| TEXAS INSTRUMENTS INCORPORATED
| Standard Linear and Logic Group
| IBIS Model of PCA9546A
| 4-CHANNEL I2C AND SMBus SWITCH WITH RESET FUNCTION
| This file contains package information for the following:
|  QFN 16-pin (RGY) package as [Component] PCA9546A_RGY
|  SOIC 16-pin (D) package as [Component] PCA9546A_D
|  SOIC 16-pin (DW) package as [Component] PCA9546A_DW
|  TSSOP 16-pin (PW) package as [Component] PCA9546A_PW
|  TVSOP 16-pin (DGV) package as [Component] PCA9546A_DGV
| This device can be powered at the following Vccs:
|  5 volt Vcc
|  3.3 volt Vcc
|  2.5 volt Vcc
| This file provides unique models under the [Model Selector] for each Vcc.
| For operation at a specific Vcc, select the appropriate model after each
| [Model Selector] keyword.
[IBIS Ver]   3.2
[Comment char]  |_char
[File Name]   pca9546a.ibs
[File Rev]   1.1 | a_die
[Date]   May 2, 2007
[Source]   Data created from TI-SPICE simulations at TI-SLL.
[Notes]   The following is an IBIS list for the PCA9546A.
   Please contact sllibis@ti.com with questions and
   comments concerning SLL IBIS models.
   - FILE REV HISTORY
   - 1.1 Release IBIS file on 5/4/07
   - Power clamp data has been deleted in all models except
   SDA terminator models as there is no power-clamp diode.
   - Non-monotonic data due to FET characteristics.
[Disclaimer] Property of Texas Instruments Incorporated.  Unauthorized
   reproduction and/or distribution is strictly prohibited.
   This product is protected under copyright law.
   Created  2007, (C) Copyright  2007, Texas Instruments
   Incorporated, All Rights Reserved
   UNLESS THERE IS A SIGNED, WRITTEN AGREEMENT TO THE
   CONTRARY, TEXAS INSTRUMENTS (TI) IS PROVIDING THE IBIS
   MODELS  AND WITHOUT ANY WARRANTY, EXPRESSED OR
   IMPLIED.  TI assumes no liability for:
   1) the accuracy of the IBIS models provided to your
   company;
   2) the proper functioning of these IBIS Models in your
   design or for any resulting applications; or
   3) infringement of patents, copyrights or intellectual
   property rights resulting from your use of these IBIS
   models.
   TI provides IBIS Models as a service to our customers.
   You and your company shall not distribute, sell or give
   these models to anyone else without prior written
   permission from TI.
   TI reserves the right to make changes to our products or
   to discontinue any semiconductor product or service
   without notice, and advises our customers to obtain the
   latest version of relevant information to verify, before
   placing orders, that the information being relied on is
   current.
   Please be aware that your receipt and use of the IBIS
   information provided shall serve as acceptance of these
   terms and conditions.  If you do not accept these terms,
   you should return or destroy the IBIS models and any
   other accompanying information immediately.
| Component PCA9546A_RGY 16-PIN QFN
[Component]   PCA9546A_RGY
[Manufacturer]   Texas Instruments, Inc.
[Package]
|   typ   min   max
R_pkg   3.900e-02   3.700e-02   4.200e-02
L_pkg   8.860e-10   8.430e-10   9.330e-10
C_pkg   3.270e-13   3.140e-13   3.360e-13
[Pin]   signal_name   model_name   R_pin   L_pin   C_pin
1   A0   PCA9546_A   4.100e-02   9.250e-10   3.140e-13
2   A1   PCA9546_A   4.000e-02   9.000e-10   3.260e-13
3   NRESET   NC   3.900e-02   8.820e-10   3.330e-13
4   SD0   PCA9546_SDX   4.100e-02   9.150e-10   3.300e-13
5   SC0   PCA9546_SCX   4.000e-02   9.000e-10   3.300e-13
6   SD1   PCA9546_SDX   4.000e-02   8.910e-10   3.290e-13
7   SC1   PCA9546_SCX   4.100e-02   9.240e-10   3.300e-13
8   GND   GND   4.200e-02   9.330e-10   3.360e-13
9   SD2   PCA9546_SDX   3.900e-02   8.850e-10   3.250e-13
10   SC2   PCA9546_SCX   3.700e-02   8.430e-10   3.210e-13
11   SD3   PCA9546_SDX   3.900e-02   8.730e-10   3.310e-13
12   SC3   PCA9546_SCX   3.800e-02   8.550e-10   3.250e-13
13   A2   PCA9546_A   3.800e-02   8.530e-10   3.260e-13
14   SCL   PCA9546_SCL   3.800e-02   8.570e-10   3.270e-13
15   SDA   PCA9546_SDA   3.800e-02   8.540e-10   3.250e-13
16   VCC   POWER   3.900e-02   8.850e-10   3.190e-13
| Component PCA9546A_D 16-PIN SOIC
[Component]   PCA9546A_D
[Manufacturer]   Texas Instruments, Inc.
[Package]
|   typ   min   max
R_pkg   3.900e-02   2.800e-02   4.900e-02
L_pkg   3.453e-09   2.350e-09   4.375e-09
C_pkg   5.210e-13   2.540e-13   7.080e-13
[Pin]   signal_name   model_name   R_pin   L_pin   C_pin
1   A0   PCA9546_A   4.200e-02   4.336e-09   7.030e-13
2   A1   PCA9546_A   4.900e-02   3.778e-09   6.340e-13
3   NRESET   NC   2.800e-02   3.449e-09   5.180e-13
4   SD0   PCA9546_SDX   2.900e-02   2.393e-09   2.540e-13
5   SC0   PCA9546_SCX   2.800e-02   2.350e-09   2.640e-13
6   SD1   PCA9546_SDX   4.800e-02   3.312e-09   4.830e-13
7   SC1   PCA9546_SCX   4.300e-02   3.629e-09   6.040e-13
8   GND   GND   4.400e-02   4.375e-09   7.080e-13
9   SD2   PCA9546_SDX   4.200e-02   4.336e-09   7.030e-13
10   SC2   PCA9546_SCX   4.900e-02   3.778e-09   6.340e-13
11   SD3   PCA9546_SDX   2.800e-02   3.449e-09   5.180e-13
12   SC3   PCA9546_SCX   2.900e-02   2.393e-09   2.550e-13
13   A2   PCA9546_A   2.800e-02   2.350e-09   2.640e-13
14   SCL   PCA9546_SCL   4.800e-02   3.312e-09   4.830e-13
15   SDA   PCA9546_SDA   4.300e-02   3.629e-09   6.040e-13
16   VCC   POWER   4.400e-02   4.375e-09   7.080e-13
| Component PCA9546A_DW 16-PIN SOIC
[Component]   PCA9546A_DW
[Manufacturer]   Texas Instruments, Inc.
[Package]
|   typ   min   max
R_pkg   4.600e-02   3.400e-02   5.700e-02
L_pkg   4.858e-09   3.987e-09   6.214e-09
C_pkg   7.150e-13   5.020e-13   1.046e-12
[Pin]   signal_name   model_name   R_pin   L_pin   C_pin
1   A0   PCA9546_A   5.700e-02   6.214e-09   1.026e-12
2   A1   PCA9546_A   5.500e-02   5.236e-09   8.180e-13
3   NRESET   NC   3.400e-02   3.987e-09   7.230e-13
4   SD0   PCA9546_SDX   3.600e-02   3.996e-09   7.260e-13
5   SC0   PCA9546_SCX   3.600e-02   3.996e-09   7.260e-13
6   SD1   PCA9546_SDX   3.400e-02   3.987e-09   7.040e-13
7   SC1   PCA9546_SCX   5.500e-02   5.236e-09   8.180e-13
8   GND   GND   5.700e-02   6.214e-09   1.046e-12
9   SD2   PCA9546_SDX   5.700e-02   6.214e-09   8.270e-13
10   SC2   PCA9546_SCX   5.500e-02   5.236e-09   5.970e-13
11   SD3   PCA9546_SDX   3.400e-02   3.987e-09   5.020e-13
12   SC3   PCA9546_SCX   3.600e-02   3.996e-09   5.050e-13
13   A2   PCA9546_A   3.600e-02   3.996e-09   5.050e-13
14   SCL   PCA9546_SCL   3.400e-02   3.987e-09   5.020e-13
15   SDA   PCA9546_SDA   5.500e-02   5.236e-09   5.970e-13
16   VCC   POWER   5.700e-02   6.214e-09   8.270e-13
| Component PCA9546A_PW 16-PIN TSSOP
[Component]   PCA9546A_PW
[Manufacturer]   Texas Instruments, Inc.
[Package]
|   typ   min   max
R_pkg   4.500e-02   3.800e-02   5.100e-02
L_pkg   2.593e-09   2.447e-09   3.080e-09
C_pkg   2.810e-13   2.430e-13   3.770e-13
[Pin]   signal_name   model_name   R_pin   L_pin   C_pin
1   A0   PCA9546_A   4.000e-02   3.080e-09   3.770e-13
2   A1   PCA9546_A   3.800e-02   2.458e-09   2.810e-13
3   NRESET   NC   5.100e-02   2.512e-09   2.550e-13
4   SD0   PCA9546_SDX   5.100e-02   2.447e-09   2.430e-13
5   SC0   PCA9546_SCX   5.100e-02   2.447e-09   2.430e-13
6   SD1   PCA9546_SDX   5.100e-02   2.512e-09   2.550e-13
7   SC1   PCA9546_SCX   3.800e-02   2.458e-09   2.810e-13
8   GND   GND   4.000e-02   3.080e-09   3.770e-13
9   SD2   PCA9546_SDX   3.900e-02   2.832e-09   3.160e-13
10   SC2   PCA9546_SCX   3.800e-02   2.460e-09   2.790e-13
11   SD3   PCA9546_SDX   5.100e-02   2.512e-09   2.550e-13
12   SC3   PCA9546_SCX   5.100e-02   2.447e-09   2.430e-13
13   A2   PCA9546_A   5.100e-02   2.447e-09   2.430e-13
14   SCL   PCA9546_SCL   5.100e-02   2.512e-09   2.550e-13
15   SDA   PCA9546_SDA   3.800e-02   2.459e-09   2.790e-13
16   VCC   POWER   3.900e-02   2.832e-09   3.160e-13
| Component PCA9546A_DGV 16-PIN TVSOP
[Component]   PCA9546A_DGV
[Manufacturer]   Texas Instruments, Inc.
[Package]
|   typ   min   max
R_pkg   3.900e-02   3.300e-02   4.500e-02
L_pkg   2.543e-09   2.320e-09   2.938e-09
C_pkg   3.860e-13   3.340e-13   4.490e-13
[Pin]   signal_name   model_name   R_pin   L_pin   C_pin
1   A0   PCA9546_A   3.500e-02   2.907e-09   4.170e-13
2   A1   PCA9546_A   4.200e-02   2.558e-09   4.460e-13
3   NRESET   NC   3.800e-02   2.341e-09   3.450e-13
4   SD0   PCA9546_SDX   3.800e-02   2.320e-09   3.340e-13
5   SC0   PCA9546_SCX   3.900e-02   2.322e-09   3.340e-13
6   SD1   PCA9546_SDX   3.800e-02   2.353e-09   3.420e-13
7   SC1   PCA9546_SCX   4.000e-02   2.536e-09   4.410e-13
8   GND   GND   3.300e-02   2.897e-09   4.180e-13
9   SD2   PCA9546_SDX   3.500e-02   2.927e-09   4.190e-13
10   SC2   PCA9546_SCX   4.500e-02   2.632e-09   4.490e-13
11   SD3   PCA9546_SDX   3.900e-02   2.368e-09   3.470e-13
12   SC3   PCA9546_SCX   3.900e-02   2.330e-09   3.350e-13
13   A2   PCA9546_A   3.900e-02   2.320e-09   3.350e-13
14   SCL   PCA9546_SCL   3.900e-02   2.361e-09   3.450e-13
15   SDA   PCA9546_SDA   4.100e-02   2.573e-09   4.460e-13
16   VCC   POWER   3.500e-02   2.938e-09   4.200e-13
[Series Switch Groups]
| Function Group States
On  1 /   | SDA/SCL<->SD/SC0
On  2 /   | SDA/SCL<->SD/SC1
On  3 /   | SDA/SCL<->SD/SC2
On  4 /   | SDA/SCL<->SD/SC3
[Series Pin Mapping]   pin_2   model_name   function_table_group
4   15   PCA9546_SDX_50_S   1
| 4   15   PCA9546_SDX_33_S   1
| 4   15   PCA9546_SDX_25_S   1
15   4   PCA9546_SDA_50_S   1
| 15   4   PCA9546_SDA_33_S   1
| 15   4   PCA9546_SDA_25_S   1
5   14   PCA9546_SCX_50_S   1
| 5   14   PCA9546_SCX_33_S   1
| 5   14   PCA9546_SCX_25_S   1
14   5   PCA9546_SCL_50_S   1
| 14   5   PCA9546_SCL_33_S   1
| 14   5   PCA9546_SCL_25_S   1
6   15   PCA9546_SDX_50_S   2
| 6   15   PCA9546_SDX_33_S   2
| 6   15   PCA9546_SDX_25_S   2
15   6   PCA9546_SDA_50_S   2
| 15   6   PCA9546_SDA_33_S   2
| 15   6   PCA9546_SDA_25_S   2
7   14   PCA9546_SCX_50_S   2
| 7   14   PCA9546_SCX_33_S   2
| 7   14   PCA9546_SCX_25_S   2
14   7   PCA9546_SCL_50_S   2
| 14   7   PCA9546_SCL_33_S   2
| 14   7   PCA9546_SCL_25_S   2
9   15   PCA9546_SDX_50_S   3
| 9   15   PCA9546_SDX_33_S   3
| 9   15   PCA9546_SDX_25_S   3
15   9   PCA9546_SDA_50_S   3
| 15   9   PCA9546_SDA_33_S   3
| 15   9   PCA9546_SDA_25_S   3
10   14   PCA9546_SCX_50_S   3
| 10   14   PCA9546_SCX_33_S   3
| 10   14   PCA9546_SCX_25_S   3
14   10   PCA9546_SCL_50_S   3
| 14   10   PCA9546_SCL_33_S   3
| 14   10   PCA9546_SCL_25_S   3
11   15   PCA9546_SDX_50_S   4
| 11   15   PCA9546_SDX_33_S   4
| 11   15   PCA9546_SDX_25_S   4
15   11   PCA9546_SDA_50_S   4
| 15   11   PCA9546_SDA_33_S   4
| 15   11   PCA9546_SDA_25_S   4
12   14   PCA9546_SCX_50_S   4
| 12   14   PCA9546_SCX_33_S   4
| 12   14   PCA9546_SCX_25_S   4
14   12   PCA9546_SCL_50_S   4
| 14   12   PCA9546_SCL_33_S   4
| 14   12   PCA9546_SCL_25_S   4
| Model PCA9546_A
[Model Selector]   PCA9546_A
PCA9546_A_50   5 volt Vcc
PCA9546_A_33   3.3 volt Vcc
PCA9546_A_25   2.5 volt Vcc
| Model PCA9546_SDX
[Model Selector]   PCA9546_SDX
PCA9546_SDX_50   5 volt Vcc
PCA9546_SDX_33   3.3 volt Vcc
PCA9546_SDX_25   2.5 volt Vcc
| Model PCA9546_SDX_S
[Model Selector]   PCA9546_SDX_S
PCA9546_SDX_50_S   5 volt Vcc
PCA9546_SDX_33_S   3.3 volt Vcc
PCA9546_SDX_25_S   2.5 volt Vcc
| Model PCA9546_SCL
[Model Selector]   PCA9546_SCL
PCA9546_SCL_50   5 volt Vcc
PCA9546_SCL_33   3.3 volt Vcc
PCA9546_SCL_25   2.5 volt Vcc
| Model PCA9546_SCL_S
[Model Selector]   PCA9546_SCL_S
PCA9546_SCL_50_S   5 volt Vcc
PCA9546_SCL_33_S   3.3 volt Vcc
PCA9546_SCL_25_S   2.5 volt Vcc
| Model PCA9546_SDA
[Model Selector]   PCA9546_SDA
PCA9546_SDA_50   5 volt Vcc
PCA9546_SDA_33   3.3 volt Vcc
PCA9546_SDA_25   2.5 volt Vcc
| Model PCA9546_SDA_S
[Model Selector]   PCA9546_SDA_S
PCA9546_SDA_50_S   5 volt Vcc
PCA9546_SDA_33_S   3.3 volt Vcc
PCA9546_SDA_25_S   2.5 volt Vcc
| Model PCA9546_SCX
[Model Selector]   PCA9546_SCX
PCA9546_SCX_50   5 volt Vcc
PCA9546_SCX_33   3.3 volt Vcc
PCA9546_SCX_25   2.5 volt Vcc
| Model PCA9546_SCX_S
[Model Selector]   PCA9546_SCX_S
PCA9546_SCX_50_S   5 volt Vcc
PCA9546_SCX_33_S   3.3 volt Vcc
PCA9546_SCX_25_S   2.5 volt Vcc
[Model]   PCA9546_SDX_50_S
Model_type  Series_switch
| variable   typ   min   max
C_comp   0   0   0
[Temperature Range]   40   100   -40
| Ambient temperature   25   85   -40
[Voltage range]   5   4.5   5.5
[On]
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[Off]
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[Model]   PCA9546_SDX_33_S
Model_type  Series_switch
| variable   typ   min   max
C_comp   0   0   0
[Temperature Range]   40   100   -40
| Ambient temperature   25   85   -40
[Voltage range]   3.3   3   3.6
[On]
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[Off]
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[Model]   PCA9546_SDX_25_S
Model_type  Series_switch
| variable   typ   min   max
C_comp   0   0   0
[Temperature Range]   40   100   -40
| Ambient temperature   25   85   -40
[Voltage range]   2.5   2.3   2.7
[On]
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[Off]
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[Model]   PCA9546_SCL_50_S
Model_type  Series_switch
| variable   typ   min   max
C_comp   0   0   0
[Temperature Range]   40   100   -40
| Ambient temperature   25   85   -40
[Voltage range]   5   4.5   5.5
[On]
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[Off]
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[Model]   PCA9546_SCL_33_S
Model_type  Series_switch
| variable   typ   min   max
C_comp   0   0   0
[Temperature Range]   40   100   -40
| Ambient temperature   25   85   -40
[Voltage range]   3.3   3   3.6
[On]
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[Off]
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[Model]   PCA9546_SCL_25_S
Model_type  Series_switch
| variable   typ   min   max
C_comp   0   0   0
[Temperature Range]   40   100   -40
| Ambient temperature   25   85   -40
[Voltage range]   2.5   2.3   2.7
[On]
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[Off]
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[Model]   PCA9546_SDA_50_S
Model_type  Series_switch
| variable   typ   min   max
C_comp   0   0   0
[Temperature Range]   40   100   -40
| Ambient temperature   25   85   -40
[Voltage range]   5   4.5   5.5
[On]
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[Off]
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[Model]   PCA9546_SDA_33_S
Model_type  Series_switch
| variable   typ   min   max
C_comp   0   0   0
[Temperature Range]   40   100   -40
| Ambient temperature   25   85   -40
[Voltage range]   3.3   3   3.6
[On]
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[Off]
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[Model]   PCA9546_SDA_25_S
Model_type  Series_switch
| variable   typ   min   max
C_comp   0   0   0
[Temperature Range]   40   100   -40
| Ambient temperature   25   85   -40
[Voltage range]   2.5   2.3   2.7
[On]
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[Off]
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[Model]   PCA9546_SCX_50_S
Model_type  Series_switch
| variable   typ   min   max
C_comp   0   0   0
[Temperature Range]   40   100   -40
| Ambient temperature   25   85   -40
[Voltage range]   5   4.5   5.5
[On]
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[Off]
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[Model]   PCA9546_SCX_33_S
Model_type  Series_switch
| variable   typ   min   max
C_comp   0   0   0
[Temperature Range]   40   100   -40
| Ambient temperature   25   85   -40
[Voltage range]   3.3   3   3.6
[On]
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[Off]
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[Model]   PCA9546_SCX_25_S
Model_type  Series_switch
| variable   typ   min   max
C_comp   0   0   0
[Temperature Range]   40   100   -40
| Ambient temperature   25   85   -40
[Voltage range]   2.5   2.3   2.7
[On]
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[Off]
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| Models and submodels in the file (27): PCA9546_A_50 (Input), PCA9546_A_33 (Input), PCA9546_A_25 (Input), PCA9546_SDX_50_S (Series_switch), PCA9546_SDX_50 (Terminator), PCA9546_SDX_33_S (Series_switch), PCA9546_SDX_33 (Terminator), PCA9546_SDX_25_S (Series_switch), PCA9546_SDX_25 (Terminator), PCA9546_SCL_50_S (Series_switch), PCA9546_SCL_50 (Terminator), PCA9546_SCL_33_S (Series_switch), PCA9546_SCL_33 (Terminator), PCA9546_SCL_25_S (Series_switch), PCA9546_SCL_25 (Terminator), PCA9546_SDA_50_S (Series_switch), PCA9546_SDA_50 (Terminator), PCA9546_SDA_33_S (Series_switch), PCA9546_SDA_33 (Terminator), PCA9546_SDA_25_S (Series_switch), PCA9546_SDA_25 (Terminator), PCA9546_SCX_50_S (Series_switch), PCA9546_SCX_50 (Terminator), PCA9546_SCX_33_S (Series_switch), PCA9546_SCX_33 (Terminator), PCA9546_SCX_25_S (Series_switch), PCA9546_SCX_25 (Terminator)
